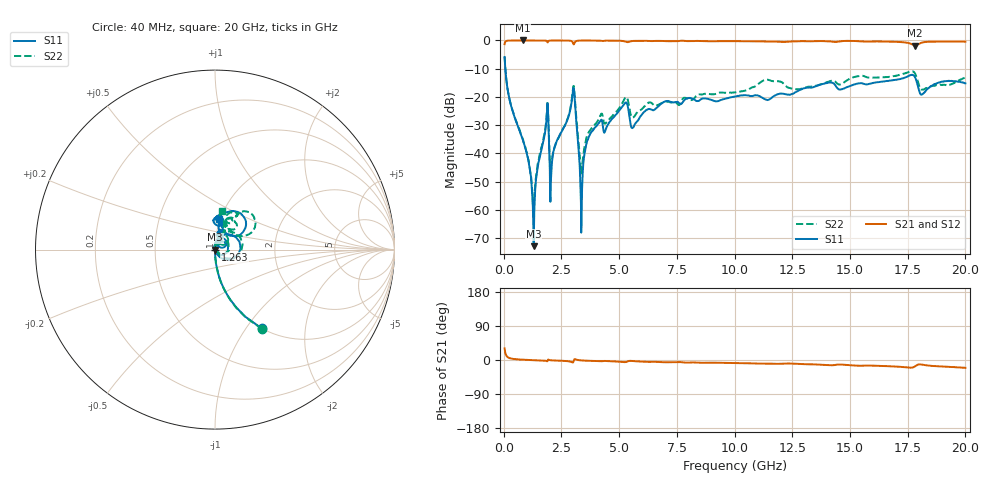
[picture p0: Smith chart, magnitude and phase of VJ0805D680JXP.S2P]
! VJ0805D680JXP
! DATE 10/29/2021  12:53
! CAPACITORS MOUNTED IN SERIES ON 25 MIL THICK MICROSTRIP SUBSTRATE
# GHz  S  MA  R  50.00
!  FREQ  S11M  S11A  S21M  S21A  S12M  S12A  S22M  S22A
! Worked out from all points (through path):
!   1601 points, 40 MHz to 20 GHz, reference 50 ohm
!   highest |S21| = 0.00 dB at 825.9 MHz (marker M1); lowest = -1.8 dB at 17.82 GHz (marker M2)
!   group delay of S21, straight-line fit = 2.9 ps
!   lowest |S11| = -72.8 dB at 1.3 GHz (marker M3), VSWR 1.00, Z = 50 + j0.0119 ohm
!   |S11| at or under -10 dB: 71.19 MHz to end of sweep
!   |S22| runs from -59.8 to -5.8 dB; largest |S21 - S12| = 0.0094
!   S11 on the Smith chart (normalised r, x): 40 MHz: 1.00, -1.19; 1.263 GHz: 1.00, -0.00; 20 GHz: 0.98, +0.35
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0.04  0.5099 -59.4  0.8594 30.6  0.8589 30.7  0.5134 -59.4
0.2895  0.07753 -85.8  0.9956 4.4  0.9968 4.3  0.07877 -85.7
0.825925  0.01732 -89.2  1 0.8  0.9995 0.7  0.01813 -87.6
1.0879  0.006713 -92.4  0.999 0.1  0.9993 0.0  0.007072 -81.6
1.26255  0.001173 -86.3  0.9986 -0.3  0.9988 -0.3  0.0012 -30.7
1.299975  0.000228 31.5  0.9993 -0.4  0.9986 -0.4  0.001332 16.3
1.8364  0.03308 71.0  0.9903 -2.4  0.9909 -2.5  0.03543 74.5
2.0859  0.006616 94.7  0.998 -0.9  0.9976 -1.0  0.007366 55.3
2.996575  0.1239 41.5  0.9145 -6.6  0.9144 -6.6  0.1339 48.5
3.10885  0.05849 -53.4  0.9577 1.9  0.9574 1.8  0.06704 -41.5
3.370825  0.0005647 77.3  0.9967 -1.1  0.9971 -1.2  0.004435 31.4
3.6328  0.01712 102.6  0.9971 -1.9  0.9979 -2.1  0.02175 84.1
4.144275  0.03558 82.2  0.993 -3.2  0.9931 -3.3  0.04278 78.1
5.2795  0.07937 48.0  0.9515 -5.5  0.9518 -5.6  0.09836 58.4
5.591375  0.02841 47.7  0.9781 -2.7  0.9779 -2.8  0.04306 50.9
6.70165  0.06794 77.4  0.9819 -5.2  0.9808 -5.3  0.07293 64.5
10.02  0.1015 77.7  0.9726 -8.0  0.9715 -8.3  0.1202 64.3
13.35083  0.1467 81.0  0.9693 -11.3  0.9691 -11.6  0.1526 66.7
16.68165  0.1933 83.0  0.9535 -16.4  0.9528 -16.7  0.2267 57.4
17.81687  0.2248 39.4  0.8136 -16.8  0.8143 -17.1  0.2612 30.9
18.11628  0.1103 54.3  0.9154 -12.3  0.914 -12.5  0.1351 45.2
20  0.1738 82.8  0.9515 -20.6  0.9512 -21.0  0.2202 79.4
